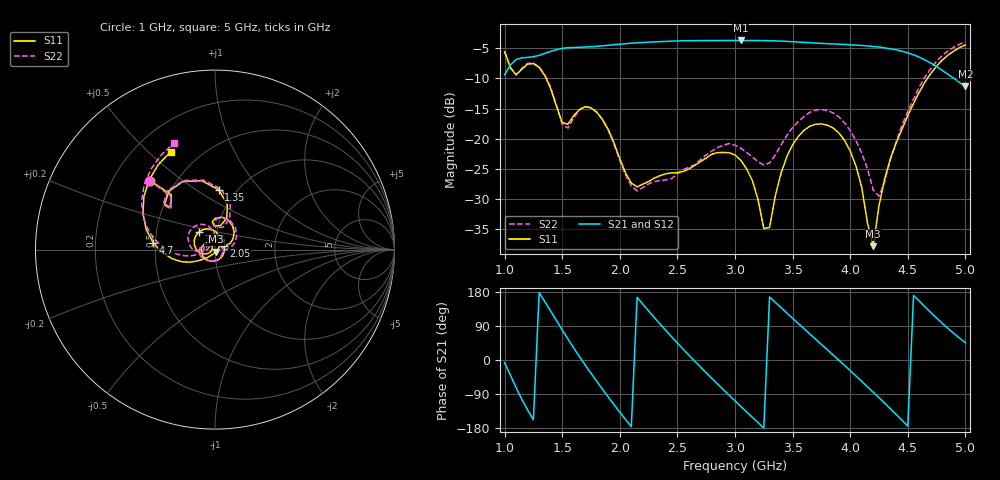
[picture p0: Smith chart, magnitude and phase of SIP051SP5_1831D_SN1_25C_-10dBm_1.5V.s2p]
# GHz  S  dB  R  50
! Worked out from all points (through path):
!   81 points, 1 GHz to 5 GHz, reference 50 ohm
!   highest |S21| = -3.72 dB at 3.05 GHz (marker M1); lowest = -11.3 dB at 5 GHz (marker M2)
!   lowest |S11| = -37.8 dB at 4.2 GHz (marker M3), VSWR 1.03, Z = 50.4 - j1.24 ohm
!   |S11| at or under -10 dB: 1.36 GHz to 4.671 GHz (3.31 GHz wide, 110 % of centre)
!   |S22| runs from -29.5 to -3.9 dB; largest |S21 - S12| = 0.005
!   S11 on the Smith chart (normalised r, x): 1 GHz: 0.36, +0.38; 1.35 GHz: 0.83, +0.62; 2.05 GHz: 1.10, +0.04; 3.75 GHz: 0.82, +0.16; 4.7 GHz: 0.49, +0.04; 5 GHz: 0.35, +0.59
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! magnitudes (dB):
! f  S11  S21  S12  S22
! 1 GHz  -5.6  -9.4  -9.4  -5.5
! 1.1 GHz  -9.4  -6.9  -6.9  -9.4
! 1.35 GHz  -9.6  -5.9  -5.9  -9.4
! 1.5 GHz  -17.3  -5.0  -5.0  -17.6
! 1.7 GHz  -14.7  -4.8  -4.8  -14.6
! 1.85 GHz  -16.8  -4.6  -4.6  -16.8
! 2.05 GHz  -25.7  -4.3  -4.3  -26.0
! 2.35 GHz  -26.1  -3.9  -3.9  -26.9
! 3 GHz  -22.7  -3.7  -3.7  -21.1
! 3.05 GHz  -23.5  -3.7  -3.7  -21.6
! 3.15 GHz  -26.9  -3.7  -3.7  -23.0
! 3.25 GHz  -34.8  -3.7  -3.7  -24.3
! 3.3 GHz  -34.7  -3.8  -3.8  -24.0
! 3.45 GHz  -22.9  -3.9  -3.9  -19.4
! 3.7 GHz  -17.6  -4.2  -4.2  -15.2
! 3.75 GHz  -17.5  -4.2  -4.2  -15.2
! 4 GHz  -22.0  -4.4  -4.4  -18.6
! 4.2 GHz  -37.8  -4.7  -4.7  -28.5
! 4.25 GHz  -31.1  -4.8  -4.8  -29.5
! 4.35 GHz  -23.2  -5.1  -5.1  -23.4
! 4.7 GHz  -9.2  -7.5  -7.4  -8.3
! 5 GHz  -4.5  -11.3  -11.3  -3.9
